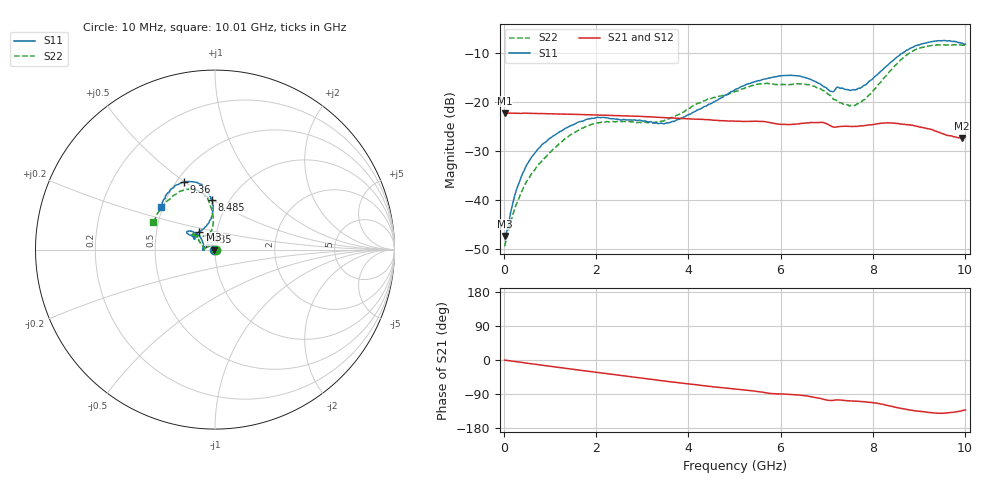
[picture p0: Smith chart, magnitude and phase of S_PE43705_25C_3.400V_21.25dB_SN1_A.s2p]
! Device ID: PE43705
! Serial: 1
! Insertion: A
! Impedance: 50 ohm
! Temp: 25C
! VDD: 3.400V
! Attenuation Step: 21.25dB
#  Hz  S  RI  R  50
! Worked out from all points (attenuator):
!   401 points, 10 MHz to 10.01 GHz, reference 50 ohm
!   highest |S21| = -22.31 dB at 10 MHz (marker M1); lowest = -27.4 dB at 9.935 GHz (marker M2)
!   lowest |S11| = -47.3 dB at 10 MHz (marker M3), VSWR 1.01, Z = 49.6 + j0.0477 ohm
!   |S11| at or under -10 dB: start of sweep to 8.664 GHz
!   |S22| runs from -49.4 to -8.4 dB; largest |S21 - S12| = 0.0008
!   S11 on the Smith chart (normalised r, x): 10 MHz: 0.99, +0.00; 7.435 GHz: 0.82, +0.16; 8.485 GHz: 0.83, +0.49; 9.36 GHz: 0.55, +0.50; 10.01 GHz: 0.49, +0.27
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1e7  -0.00428 0.000481  0.0767 -0.000326  0.0768 -0.000313  0.00337 0.000343
6e7  -0.00409 0.00259  0.0765 -0.00152  0.0765 -0.00144  0.00367 0.00191
2.85e8  -0.00604 0.012  0.0759 -0.00646  0.0759 -0.00641  0.00158 0.00934
5.6e8  -0.0133 0.0219  0.0748 -0.0124  0.0749 -0.0125  -0.00515 0.0165
1.01e9  -0.033 0.0274  0.072 -0.0218  0.0721 -0.0217  -0.0244 0.0188
1.685e9  -0.0607 0.0172  0.0655 -0.0342  0.0656 -0.0342  -0.0527 0.00886
2.185e9  -0.0686 0.00311  0.0593 -0.0422  0.0593 -0.0422  -0.0618 -0.00125
3.36e9  -0.0597 0.00412  0.0409 -0.0559  0.0409 -0.0559  -0.0616 0.00863
3.835e9  -0.0623 0.0256  0.0329 -0.0589  0.033 -0.0589  -0.0719 0.026
5.01e9  -0.0996 0.0875  0.0148 -0.0615  0.015 -0.0616  -0.1042 0.0728
5.535e9  -0.1292 0.1004  0.00678 -0.0625  0.00693 -0.0626  -0.1216 0.0892
6.01e9  -0.1524 0.1019  0.000613 -0.0588  0.000708 -0.0587  -0.1203 0.0888
6.685e9  -0.1433 0.0822  -0.00787 -0.0608  -0.0078 -0.0607  -0.1202 0.0799
7.085e9  -0.1098 0.0652  -0.0164 -0.0543  -0.0163 -0.0542  -0.0849 0.0779
7.435e9  -0.0909 0.097  -0.0168 -0.0536  -0.0166 -0.0539  -0.0496 0.0792
7.785e9  -0.0449 0.1367  -0.0193 -0.0534  -0.019 -0.0536  -0.0243 0.1002
8.36e9  -0.0108 0.2443  -0.0313 -0.0522  -0.0312 -0.0522  -0.0137 0.2012
8.485e9  -0.0168 0.2742  -0.0343 -0.0496  -0.0339 -0.05  -0.0216 0.2332
8.91e9  -0.0723 0.3601  -0.0393 -0.041  -0.0391 -0.0411  -0.0856 0.325
9.36e9  -0.1715 0.3757  -0.0386 -0.0324  -0.0387 -0.0323  -0.1843 0.3272
9.935e9  -0.2935 0.2626  -0.0296 -0.031  -0.0297 -0.031  -0.3291 0.1815
1.001e10  -0.3018 0.2384  -0.029 -0.0324  -0.0292 -0.0328  -0.3447 0.1522
